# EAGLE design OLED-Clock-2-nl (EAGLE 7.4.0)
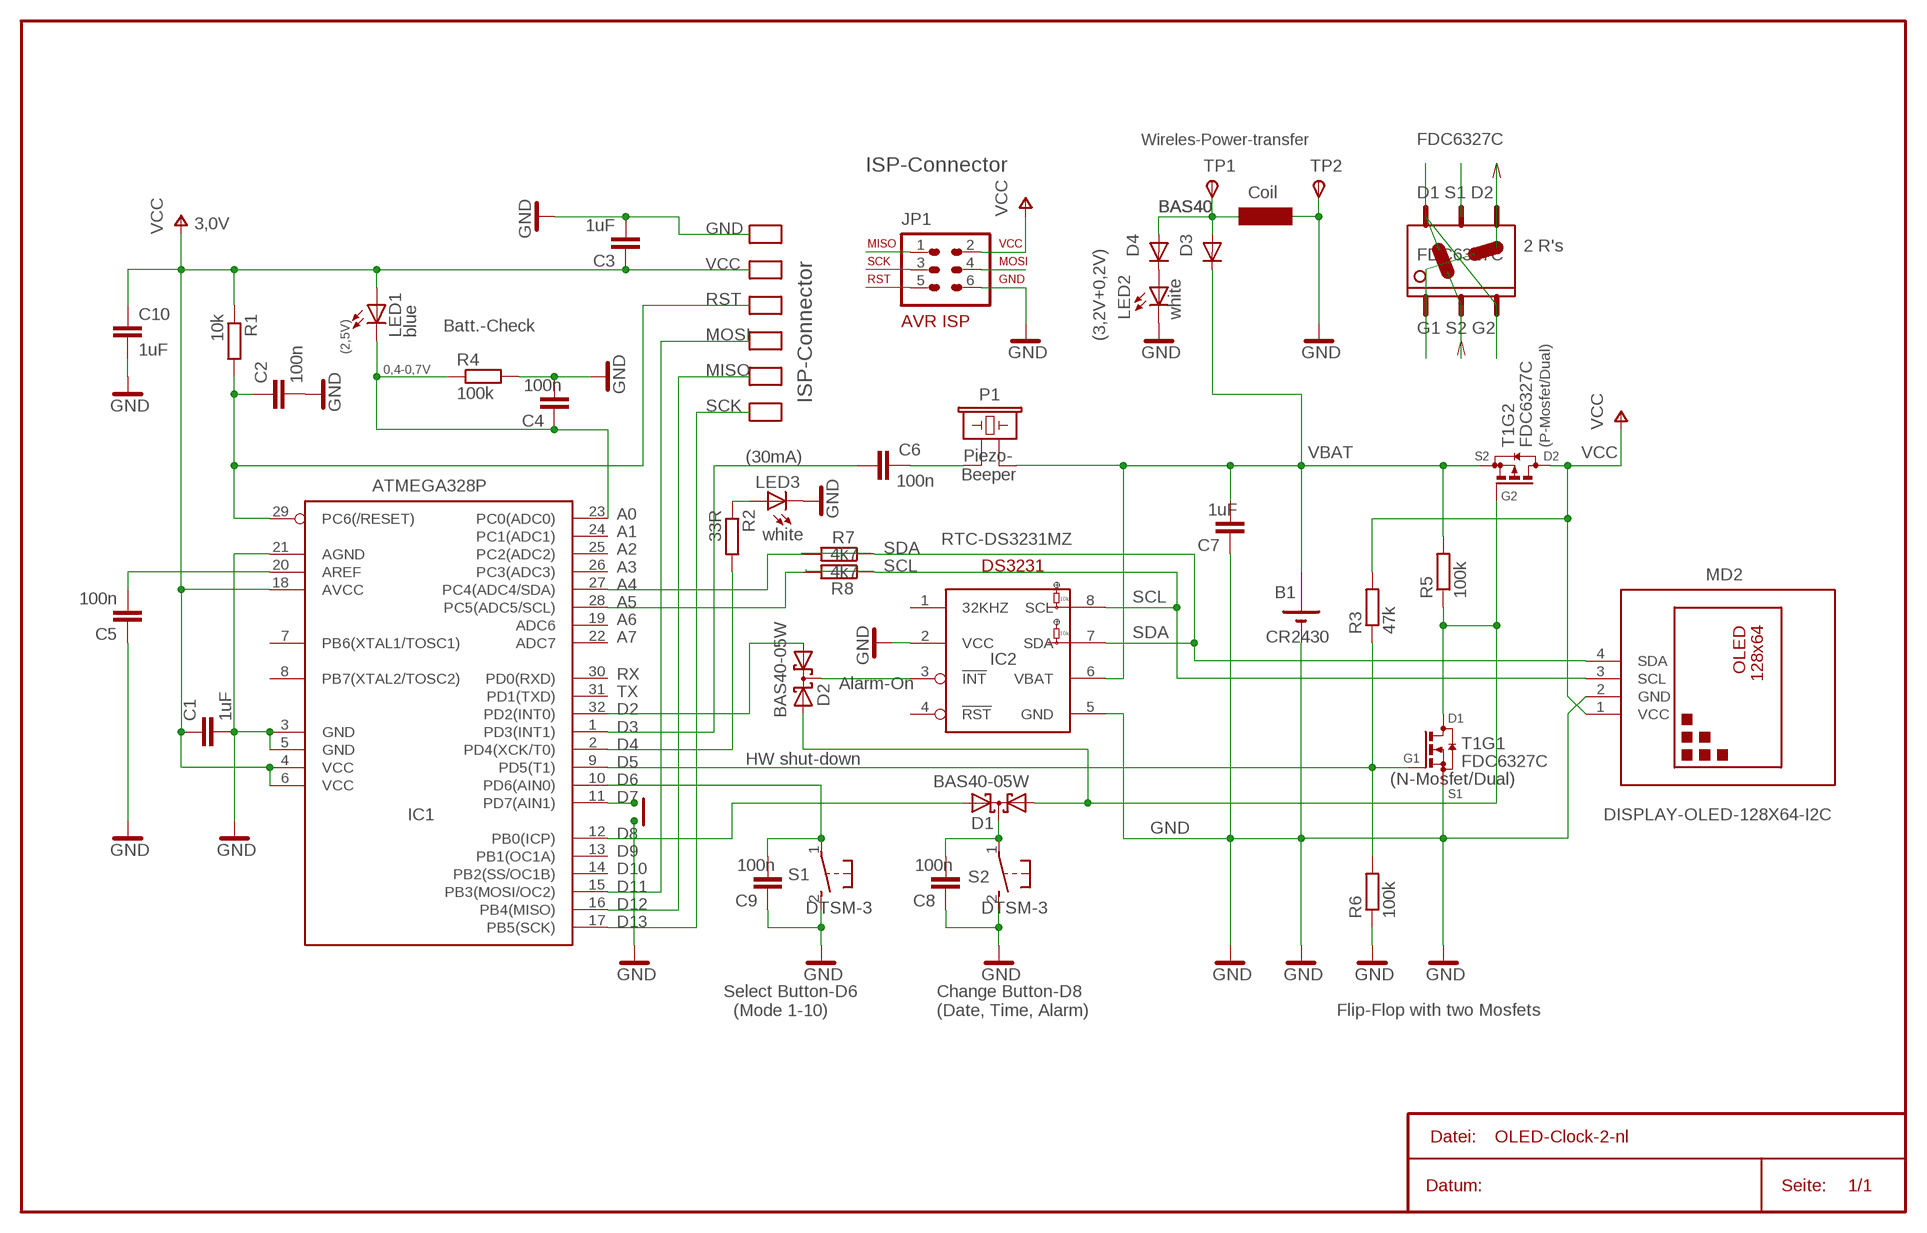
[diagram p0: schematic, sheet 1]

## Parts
C1  1uF  C-EUC0603  [C0603]
C2  100n  C-EUC0603  [C0603]
C3  1uF  C-EUC0603  [C0603]
C4  100n  C-EUC0603  [C0603]
C5  100n  C-EUC0603  [C0603]
C6  100n  C-EUC0805W  [C0805W]
C7  1uF  C-EUC0603  [C0603]
C8  100n  C-EUC0603  [C0603]
C9  100n  C-EUC0603  [C0603]
C10  1uF  C-EUC0603  [C0603]
D1  BAS40-05W  BAS40-05  [SOT323-R]
D2  BAS40-05W  BAS40-05  [SOT323-R]
D3  BAS40  DIODE-SOD523  [SOD523]
D4  BAS40  DIODE-SOD523  [SOD523]
IC1  ATMEGA328P  MEGA8-AI  [TQFP32-08]
IC2  DS3231  [SO08]
JP1  AVR-ISP-6  AVR-ISP-6VERT  [AVR-ISP-6]
LED1  blue  LEDCHIPLED_0805  [CHIPLED_0805]
LED2  white  LEDCHIPLED_0603  [CHIPLED_0603]
LED3  white  LEDCHIPLED_1206  [CHIPLED_1206]
MD2  DISPLAY-OLED-128X64-I2C  [DISPLAY-OLED-128X64-I2C]
R1  10k  R-EU_R0603  [R0603]
R2  33R  R-EU_R0603  [R0603]
R3  47k  R-EU_R0603  [R0603]
R4  100k  R-EU_R0603  [R0603]
R5  100k  R-EU_R0603  [R0603]
R6  100k  R-EU_R0603  [R0603]
R7  4k7  R-EU_R0402  [R0402]
R8  4k7  R-EU_R0402  [R0402]
S1  DTSM-3  [DTSM-3]
S2  DTSM-3  [DTSM-3]
T1  FDC6327C  NP_MOSFET_SOT23-6  [SOT23-6]
TP1  TPSB1,27  [B1,27]
TP2  TPSB1,27  [B1,27]

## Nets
BEEP: C6.1 IC1.1(PD3(INT1))
GND: C1.2 C2.2 C3.2 C4.2 C5.1 C7.1 C8.1 C9.1 C10.2 IC1.3(GND) IC1.5(GND) IC1.21(AGND) IC2.2(VCC) IC2.5(GND) JP1.6 LED2.C LED3.C MD2.2(GND) R4.2 R6.1 S1.2 S2.2 T1.5(S) TP2.TP(PP)
MISO: IC1.16(PB4(MISO)) JP1.1
MOSI: IC1.15(PB3(MOSI/OC2)) JP1.4
N$1: D1.1(A1) D2.2(A2) R5.1 T1.3(G) T1.6(D)
N$2: C9.2 IC1.10(PD6(AIN0)) S1.1
N$5: C6.2
N$6: C8.2 D1.3(C) S2.1
N$7: IC1.11(PD7(AIN1))
N$12: IC1.28(PC5(ADC5/SCL)) R8.2
N$13: C4.1 IC1.23(PC0(ADC0)) LED1.C R4.1
N$16: D1.2(A2) IC1.12(PB0(ICP))
N$21: D2.3(C) IC2.3(!INT)
N$22: LED3.A R2.1
N$23: IC1.2(PD4(XCK/T0)) R2.2
N$25: D3.A D4.A TP1.TP(PP)
N$26: IC1.9(PD5(T1)) R3.1 R6.2 T1.1(G)
N$29: D4.C LED2.A
N$32: C5.2 IC1.20(AREF)
N$33: D2.1(A1) IC1.32(PD2(INT0))
N$34: IC1.27(PC4(ADC4/SDA)) R7.2
RST: C2.1 IC1.29(PC6(/RESET)) JP1.5 R1.2
SCK: IC1.17(PB5(SCK)) JP1.3
SCL: IC2.8(SCL) MD2.3(SCL) R8.1
SDA: IC2.7(SDA) MD2.4(SDA) R7.1
VBAT: C7.2 D3.C IC2.6(VBAT) R5.2 T1.2(S)
VCC: C1.1 C3.1 C10.1 IC1.4(VCC) IC1.6(VCC) IC1.18(AVCC) JP1.2 LED1.A MD2.1(VCC) R1.1 R3.2 T1.4(D)
Unconnected: IC1.7(PB6(XTAL1/TOSC1)) IC1.8(PB7(XTAL2/TOSC2)) IC1.13(PB1(OC1A)) IC1.14(PB2(SS/OC1B)) IC1.19(ADC6) IC1.22(ADC7) IC1.24(PC1(ADC1)) IC1.25(PC2(ADC2)) IC1.26(PC3(ADC3)) IC1.30(PD0(RXD)) IC1.31(PD1(TXD)) IC2.1(32KHZ) IC2.4(!RST)

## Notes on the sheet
- Wireles-Power-transfer | FDC6327C
- ISP-Connector
- Coil | D1 S1 D2
- 3,0V
- 2 R's
- FDC6327C
- Batt.-Check | G1 S2 G2
- (3,2V+0,2V)
- (2,5V)
- 0,4-0,7V
- ISP-Connector | P1
- (P-Mosfet/Dual)
- (30mA) | Piezo- | S2 | D2
- Beeper
- G2
- RTC-DS3231MZ
- +
- B1
- 10k
- +
- 10k
- A0
  A1
  A2
  A3
  A4
  A5
  A6
  A7
- CR2430
- IC2
- Alarm-On
- D1
- HW shut-down | G1
- (N-Mosfet/Dual)
- S1
- RX
  TX
  D2
  D3
  D4
  D5
  D6
  D7
- D8
  D9
  D10
  D11
  D12
  D13
- Select Button-D6
    (Mode 1-10)
- Change Button-D8
  (Date, Time, Alarm)
- Flip-Flop with two Mosfets

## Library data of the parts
C1-C10 = rcl1:C-EU: CAPACITOR, European symbol
D1 D2 = diode1:BAS40-05: Silicon Schottky Diodes General-purpose diode for high-speed switching
D3 D4 = diode1:DIODE-: DIODE
IC1 = avr-7:MEGA8: MICROCONTROLLER 8 Kbytes FLASH 1 kbytes SRAM 512 bytes EEPROM USART 6-channel 10 bit ADC 2-channel 8 bit ADC
IC2 = DS3231:DS3231
JP1 = avr-7:AVR-ISP-6: AVR ISP-6 Serial Programming Header
LED1-LED3 = led:LED: LED
MD2 = diy-modules:DISPLAY-OLED-128X64-I2C: 128x64 Dot Matrix OLED Module based on SSD1306 chip Variant with I2C interface More details available here: http://www.instructables.com/id/Monochrome-096-i2c-OLED-display-with-arduino-SSD13/ SSD1306 datasheet: https://cdn-shop.adafruit.com/datasheets/SSD1306.pdf Click here to find device on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
R1-R8 = rcl:R-EU_: RESISTOR, European symbol
S1 S2 = switch-tact:DTSM-3
T1 = transistor-small-signal:NP_MOSFET_SOT23-6: Dual N- & P-Channel Mosfet 20V / ~2A / ~1W / ~100mO / SOT23-6
TP1 TP2 = testpad-1:TPS: TEST PIN

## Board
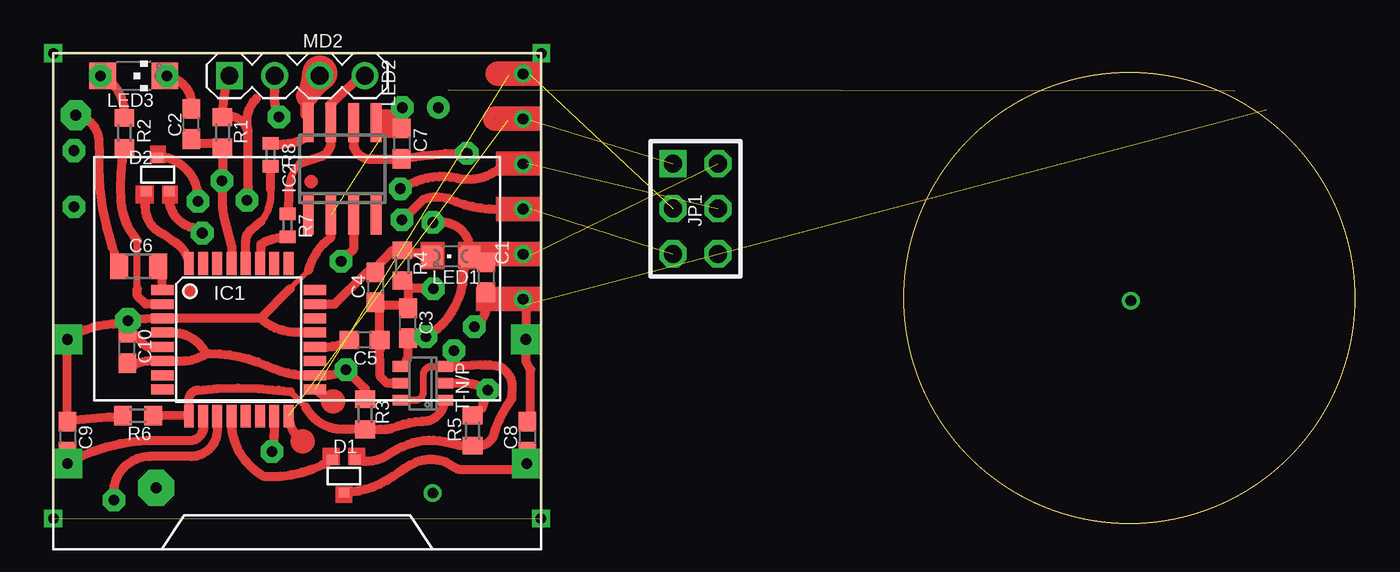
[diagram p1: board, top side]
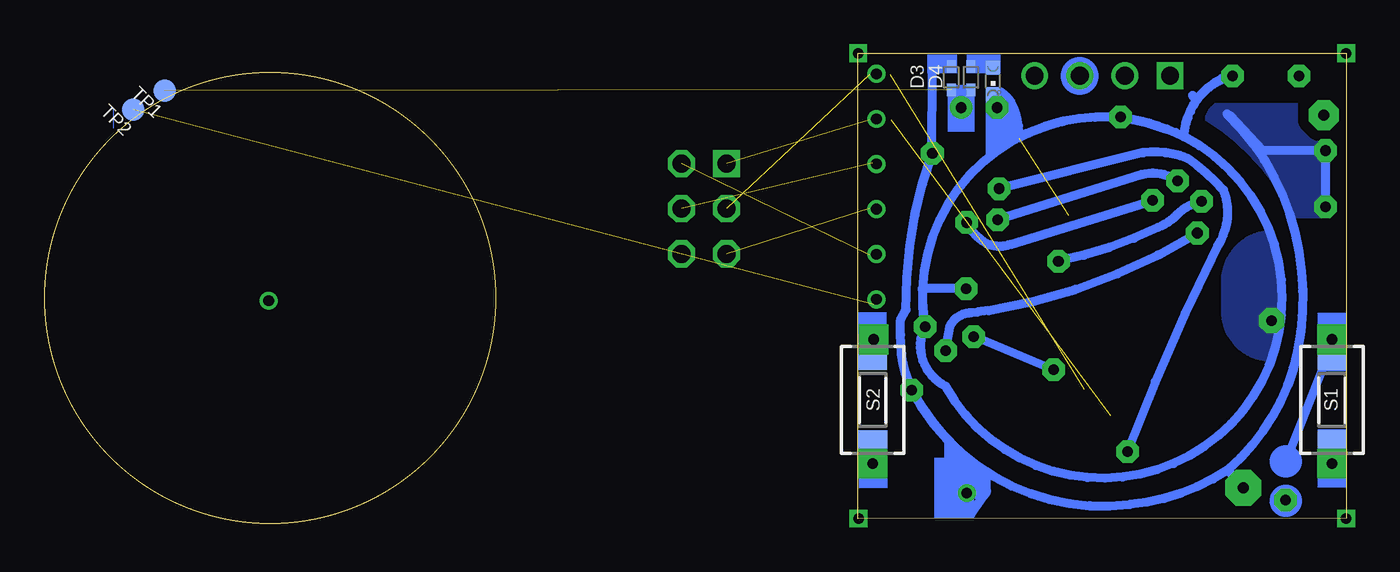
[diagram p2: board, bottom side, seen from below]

Size 73.26 x 26.47 mm. Coordinates in mm from the lower left corner, seen from the top.
Outline: 27.46,0.26 27.46,26.47 0,26.47 0,0.28 27.46,0.26
Outline: circle at 60.56,12.7 radius 12.7
Copper layers (1*16): Top 0.035mm / dielectric 1.5mm / Bottom 0.035mm
Design rules "default": minimum track width 10mil, minimum drill 24mil, track to track 8mil, track to pad 8mil, pad to pad 8mil, via to via 8mil, smd to smd 8mil, copper to edge 40mil, drill to drill 8mil, minimum pad ring 10mil, minimum via ring 8mil, stop-mask expansion 4mil, vias tented up to drill 0mil, thermal gap 10mil

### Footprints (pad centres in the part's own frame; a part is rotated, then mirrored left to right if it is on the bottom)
C0603 = smd 1.1 x 1: 1 -0.85,0; 2 0.85,0
C0805W = smd 1.016 x 1.422: 1 -1.092,0; 2 1.092,0
SOT323-R = smd 0.6 x 0.55: 1 -0.65,-0.925; 2 0.65,-0.925; 3 0,0.925
SOD523 = smd 0.7 x 0.5: A 0.7,0; C -0.6,0
TQFP32-08 = smd 1.27 x 0.559: 1 -4.293,2.8; 2 -4.293,2; 3 -4.293,1.2; 4 -4.293,0.4; 5 -4.293,-0.4; 6 -4.293,-1.2; 7 -4.293,-2; 8 -4.293,-2.8; 17 4.293,-2.8; 18 4.293,-2; 19 4.293,-1.2; 20 4.293,-0.4; 21 4.293,0.4; 22 4.293,1.2; 23 4.293,2; 24 4.293,2.8 | smd 0.559 x 1.27: 9 -2.8,-4.293; 10 -2,-4.293; 11 -1.2,-4.293; 12 -0.4,-4.293; 13 0.4,-4.293; 14 1.2,-4.293; 15 2,-4.293; 16 2.8,-4.293; 25 2.8,4.293; 26 2,4.293; 27 1.2,4.293; 28 0.4,4.293; 29 -0.4,4.293; 30 -1.2,4.293; 31 -2,4.293; 32 -2.8,4.293
SO08 = smd 0.6 x 2.2: 1 -1.905,-2.6; 2 -0.635,-2.6; 3 0.635,-2.6; 4 1.905,-2.6; 5 1.905,2.6; 6 0.635,2.6; 7 -0.635,2.6; 8 -1.905,2.6
AVR-ISP-6 = drill 1.016 square: 1 -2.54,-1.27 | drill 1.016 octagon: 2 -2.54,1.27; 3 0,-1.27; 4 0,1.27; 5 2.54,-1.27; 6 2.54,1.27
CHIPLED_0805 = smd 1.2 x 1.2: A 0,-1.05; C 0,1.05
CHIPLED_0603 = smd 0.8 x 0.8: A 0,-0.75; C 0,0.75
CHIPLED_1206 = smd 1.5 x 1.5: A 0,-1.75; C 0,1.75
DISPLAY-OLED-128X64-I2C = drill 1 square: 1 -3.81,12.7 | drill 1: 2 -1.27,12.7; 3 1.27,12.7; 4 3.81,12.7
R0603 = smd 1 x 1.1: 1 -0.85,0; 2 0.85,0
R0402 = smd 0.7 x 0.9: 1 -0.65,0; 2 0.65,0
DTSM-3 = smd 2 x 1.6: 1 -2.7,0; 2 2.7,0
SOT23-6 = smd 0.6 x 1: 1 -0.95,-1.2; 2 0,-1.2; 3 0.95,-1.2; 4 0.95,1.2; 5 0,1.2; 6 -0.95,1.2
B1,27 = smd 1.27 x 1.27: TP 0,0

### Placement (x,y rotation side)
C1  24.36,13.86 270 top
C2  7.77,22.49 90 top
C3  19.96,11.28 90 top
C4  18.13,13.3 270 top
C5  17.51,10.33 180 top
C6  4.8,14.49 180 top
C7  19.61,21.39 270 top
C8  26.67,4.88 270 top
C9  0.79,4.88 270 top
C10  4.17,9.88 90 top
D1  16.35,2.66 180 top
D2  5.87,19.65 0 top
D3  22.23,25.12 270 bottom
D4  21.11,25.12 270 bottom
IC1  10.43,10.34 0 top
IC2  16.26,19.97 0 top
JP1  36.14,17.72 270 top
LED1  22.37,15.05 90 top
LED2  19.88,24.91 180 bottom
LED3  4.52,25.2 270 top
MD2  13.72,12.51 0 top
R1  9.53,22.03 270 top
R2  4.01,21.99 270 top
R3  17.55,6.15 90 top
R4  19.63,14.53 270 top
R5  23.59,5.23 90 top
R6  4.76,6.07 0 top
R7  13.18,16.79 270 top
R8  12.22,20.76 270 top
S1  0.79,6.95 90 bottom
S2  26.64,6.95 90 bottom
T1  20.8,7.89 90 top
TP1  66.5,24.37 135 bottom
TP2  68.28,23.31 135 bottom

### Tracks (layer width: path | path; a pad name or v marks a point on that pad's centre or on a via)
BEEP
  Top 0.508: IC1.1 6.14,14.8 C6.1
GND  (via drill 0.6 pad 0.81, 0.6 pad 1.27, 0.6 pad 1.42, 0.6 pad 1.68)  (3 unrouted)
  Top 0.305: 13.34,13.22 14.37,14.25
  Top 0.508: 26.37,12.56 26.27,12.66 24.47,12.66 C1.2 24.36,12.33 arc-63 v23.69,11.07 | 26.37,12.56 26.59,12.34 v26.59,10.36 26.59,9.13 26.87,8.65 26.87,5.41 C8.1 | 18.4,9.82 C5.1 | T1.5 18.78,7.89 18.4,8.27 C5.1 | 19.86,11.97 C3.2 | 11.67,11.55 11.66,11.54 IC1.3 5.56,11.55 v4.2,11.42 | 11.67,11.55 13.34,13.22 | 14.37,14.25 arc-40 15.62,16.1 IC2.2 | 0.79,5.44 C9.1 | C9.1 v0.79,10.36 arc-36 3.76,11.23 v4.2,11.42 | IC1.21 13.73,10.76 arc-44 11.67,11.55 | IC2.5 C7.1 19.53,22.19 arc-17 v19.64,23.42 | v26.43,12.62 26.37,12.56 | 19.96,11.87 C3.2 | R4.2 19.52,13.57 19.96,13.57 19.96,13.22 | 19.96,13.22 C3.2 | v21.39,13.22 19.96,13.22 | C3.2 19.96,12.32 | 18.43,12.31 C4.2 | C5.1 18.36,12.25 18.43,12.31 | 18.43,12.31 19.77,12.31 C3.2 | v12.7,22.9 arc-28 12.46,24.33 MD2.2 v12.46,25.2 | C2.2 7.81,23.74 arc70 v6.39,25.2 LED3.C | C10.2 3.89,11.2 v4.2,11.42 | IC1.5 5.26,9.94 4.24,10.97 v4.2,11.42 | R6.1 3.81,5.97 3.06,5.97 0.83,5.77 C9.1
  Bottom 0.508: S2.2 26.59,9.51 v26.59,10.36 | S1.2 0.79,10.12 | 0.79,10.12 v0.79,10.36 | v21.39,13.22 23.85,13.22 arc-11 v23.69,11.07 23.76,11.11 23.76,11.06 | 3.65,11.71 arc-195 23.73,11.15 23.76,11.06 | 23.76,11.06 23.89,10.64 arc-78 22.54,7.74 arc-146 3.65,11.79 arc-90 3.73,11.54 v4.2,11.42 | 10.6,22.38 arc-46 18.41,21.71 arc-30 18.85,23.69 arc-31 19.45,24.29 v19.64,23.42 19.88,24.01 LED2.C | 0.79,10.12 3.41,3.45 | v12.7,22.9 12.62,22.82 arc14 10.6,22.38 | 10.6,22.38 arc10 9.13,21.79 arc65 6.67,25.2 v6.39,25.2 arc-41 8.41,23.85 8.65,24.09
  pour Bottom: 4.17,16.39 arc-84 6.91,13.93 6.91,11.79 arc-90 4.13,9.25 arc-38
MISO  (via drill 0.6 pad 0.81)  (2 unrouted)
  Top 0.508: 25.58,22.72 26.47,22.72 | 26.47,22.72 26.85,22.72 | IC1.16 13.26,5.99 arc50 13.93,4.72 | v26.43,22.78 26.43,22.76 26.47,22.72
MOSI  (via drill 0.6 pad 0.81, 0.6 pad 1.27)  (1 unrouted)
  Top 0.508: IC1.15 12.43,5.49 arc-11 v12.3,4.05 | v19.53,18.85 20.4,19.25 arc-32 22.7,19.45 arc44 24.84,19.8 arc-38 v26.43,20.24 26.63,20.24 26.67,20.28
  Bottom 0.508: v19.53,18.85 11.43,20.88 arc29 8.93,20.56 arc13 6.91,18.77 arc53 7.22,15.64 arc-6 v12.3,4.05
N$1  (via drill 0.6 pad 1.27)
  Top 0.406: T1.6 20.39,6.94 arc86 20.82,7.36 20.82,8.39 arc-79 21.26,8.84 T1.3
  Top 0.508: 22.62,8.84 T1.3 | 22.62,8.84 22.5,9.12 v22.54,9.72 | D1.1 arc46 18.69,3.77 arc-10 19.68,4.33 arc-44 22.3,4.52 22.88,4.38 R5.1 24.13,4.38 arc51 24.77,4.92 arc-18 25.8,7.02 25.84,7.6 arc68 25.08,8.85 arc16 24.05,8.93 arc1 22.62,8.84 | v8.37,16.35 7.82,16.67 arc-88 D2.2
  Bottom 0.508: v22.54,9.72 22.3,11.07 arc67 21.11,11.87 20.76,11.91 20.12,11.99 arc-22 v8.37,16.35
N$2  (via drill 0.6 pad 1.68)
  Top 0.508: v0.79,3.37 0.87,3.37 0.87,3.29 v0.79,3.37 | v0.79,3.37 C9.2 | IC1.10 8.45,5.64 arc-87 7.86,4.68 5.32,4.68 arc28 v0.79,3.37
  Bottom 0.508: S1.1 v0.79,3.37
N$4  (via drill 0.6)
  other vias: 0,26.47
N$5  (via drill 0.6 pad 1.68)
  Top 0.508: C6.2 arc-27 2.58,21.15 2.58,21.47 arc81 v1.26,22.99
N$6  (via drill 0.6 pad 1.68)
  Top 0.406: C8.2 26.64,4.03 | 26.64,4.03 S2.1 | 26.64,4.03 v26.64,3.37
  Top 0.508: D1.3 arc33 19.12,2.65 arc-12 20.4,3.45 arc-42 22.11,3.45 22.78,3.06 26.43,3.06 v26.64,3.37
  Bottom 0.406: S2.1 v26.64,3.37
N$7  (via drill 0.6 pad 1.27)
  Top 0.508: IC1.11 arc-23 9.13,4.72 arc-67 7.78,3.77 5.4,3.77 arc100 v3.41,1.31
N$9  (via drill 0.6)
  other vias: 27.46,26.47
N$10  (via drill 0.6)
  other vias: 27.44,0.28
N$11  (via drill 0.6)
  other vias: 0,0.28
N$12
  Top 0.406: 11.67,16.99 arc52 12.22,18.85
  Top 0.508: IC1.28 10.84,15.87 arc-53 11.15,16.55 11.67,16.99 | 12.22,18.85 R8.2
N$13
  Top 0.508: LED1.C 21.32,15.13 | IC1.23 15.84,12.34 17.65,14.15 C4.1 18.1,14.15 18.1,14.33 19.12,15.38 R4.1 19.63,15.24 21.04,15.24 21.04,15.13 LED1.C | LED1.C | 21.2,15.05 LED1.C
N$16
  Top 0.508: IC1.12 10.03,5.49 arc55 11.83,2.66 12.78,2.66 arc24 D1.2
N$21  (via drill 0.6 pad 1.27)
  Top 0.508: IC2.3 16.89,15.43 v16.19,14.76 | D2.3 6.02,20.68 arc-87 v8.14,18.14
  Bottom 0.508: v8.14,18.14 arc-35 9.53,17.38 arc25 10.6,16.67 arc14 v16.19,14.76
N$22  (via drill 0.6 pad 1.27)
  Top 0.508: R2.1 arc64 LED3.A v2.66,25.2
N$23
  Top 0.406: 4.72,13.22 4.72,15.91
  Top 0.508: IC1.2 5.2,12.34 4.72,12.82 4.72,13.22 | R2.2 arc14 3.81,18.18 arc34 4.72,15.91
N$24
  Top 0.406: 14.68,23.93 arc-13 15.56,24.8
N$25  (via drill 0.6 pad 1.27)  (1 unrouted)
  Bottom 0.508: D4.A D3.A 21.67,24.41 v21.67,23.42
N$26
  Top 0.356: 13.34,7.42 14.21,6.55
  Top 0.508: 13.34,7.42 12.66,7.5 arc13 8.14,7.5 arc77 7.62,7.02 IC1.9 7.61,5.83 7.62,5.83 7.52,6.12 R6.2 | 14.21,6.55 arc60 16.17,5.3 R3.1 18.4,5.3 arc19 19.05,5.36 arc-19 20.74,5.75 arc93 T1.1
N$27
  Top 0.406: 13.89,24.17 arc23 14.21,25.44
N$29
  Bottom 0.508: D4.C 20.1,25.72 LED2.A
N$30  (via drill 0.6)
  other vias: 60.64,12.54
N$31
  Bottom 0: 69.37,22.26 69.37,23.38
N$32
  Top 0.508: IC1.20 arc30 16.67,10.26 C5.2
N$33
  Top 0.508: IC1.32 arc56 6.71,15.91 6.15,16.31 arc-93 5.34,18.6 D2.1
N$34
  Top 0.508: R7.2 arc28 11.67,15.72 IC1.27
RST  (via drill 0.6 pad 0.81, 0.6 pad 1.27)  (1 unrouted)
  Top 0.508: IC1.29 10.03,15.65 9.6,17.26 arc-11 9.53,18.89 v9.48,19.29 9.53,19.33 R1.2 9.31,21.39 7.98,21.39 C2.1 | v19.61,17.11 19.68,17.11 20.84,18.26 arc-35 22.23,18.3 arc25 25,17.7 v26.43,17.7 26.83,17.74
  Bottom 0.508: v9.48,19.29 arc-51 11.51,19.65 v19.61,17.11
SCK  (via drill 0.6 pad 0.81)  (2 unrouted)
  Top 0.508: IC1.17 15.68,6.83 | 25.64,25.28 26.43,25.28 | 26.43,25.28 26.83,25.28 | v26.43,25.32 26.43,25.28
SCL  (via drill 0.6 pad 1.27)
  Top 0.508: MD2.3 v15,25.2 | 14.3,23.19 14.28,23.06 IC2.8 14.33,21.95 14.21,21.71 arc-39 R8.1
  Top 0.762: 14.28,24.06 14.28,23.06
  Top 1.27: MD2.3 14.28,24.06
SDA  (via drill 0.6 pad 1.27)
  Top 0.406: 13.89,20.28 arc50 13.26,18.77
  Top 0.508: v17.54,25.2 MD2.4 17.31,25.21 15.55,23.56 IC2.7 15.62,21.32 arc-48 15.1,20.68 13.89,20.28 | 13.26,18.77 13.26,18.3 R7.1
VBAT  (via drill 0.6 pad 0.81, 0.6 pad 1.27, 0.6 pad 2.03)
  Top 0.508: T1.2 22.79,7.89 arc-29 24.29,7.62 v24.45,7.5 24.14,6.48 R5.2 | IC2.6 16.89,21.24 arc80 18.02,20.52 19.17,20.52 C7.2 arc-12 v23.29,20.84
  Bottom 0.508: v24.45,7.5 arc24 25.08,10.64 25.08,11.47 24.77,12.03 arc21 v23.29,20.84 23.34,20.95 23.32,25.45 23.05,25.72 D3.C | 6.71,23.06 arc36 2.66,15.32 arc21 2.74,9.68 arc37 6.66,3.02 | v24.45,7.5 arc-70 12.18,1.07 arc-29 6.66,3.02 | 20.31,2.84 arc25 v24.45,7.5 | v5.79,2 6.66,3.02 | 20.32,2.04 v21.35,1.71 20.39,1.57 21.11,0.53 | v1.15,17.82 v1.15,20.99 4.68,20.99 6.55,22.98
  Bottom 0.61: 22.3,4.56 22.3,2.84 20.31,2.84 20.31,1.73 20.32,2.04
  pour Bottom (isolate 0.61): 7.86,23.53 7.86,22.82 arc32 2.9,17.34 0.24,17.34 0.24,21.27 2.62,23.53
VCC  (via drill 0.6 pad 0.81, 0.6 pad 1.27)  (1 unrouted)
  Top 0.508: R3.2 17.55,7.58 v16.47,8.65 16.38,8.58 arc-27 IC1.18 14,8.34 arc-20 11.99,8.89 arc25 8.81,9.56 8.59,9.55 | T1.4 arc52 19.96,9.43 C3.1 20.05,10.52 v20.95,10.52 21.27,10.68 arc59 23.1,14.72 LED1.A | 26.39,15.12 24.85,15.12 C1.1 23.68,14.79 LED1.A | 26.39,15.12 26.83,15.12 | IC1.4 6.9,10.74 arc-60 8.59,9.55 | 8.59,9.55 arc-32 7.2,9.14 IC1.6 5.29,9.14 4.64,8.97 4.14,8.97 C10.1 | v26.43,15.16 26.39,15.12 | LED1.A arc107 21.75,16.95 v21.35,16.95 | v10.89,18.19 10.95,19.05 10.95,22.07 | 10.95,22.07 arc96 R1.1 arc-17 9.84,25.04 v9.92,25.2 MD2.1 | 11.43,23.93 arc59 10.95,22.15 10.95,22.07
  Bottom 0.508: v16.47,8.65 v20.95,10.52 | v10.89,18.19 18.89,15.72 arc45 20.24,15.76 arc32 v21.35,16.95
(copper drawn outside any net)
  shapes: Bottom area x15, Bottom circle x3, Top area x18, Top circle x8

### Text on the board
tNames: T-N/P
tValues: Board: ~28 x 26,5 mm | Layer: | 1. Beeper (ø24mm) / 2. Batt. (CR2430) / 3. ATmega-Board / 4. OLED-Display | (GND VCC) | Coil with / 30 loops / Cu 0.1mm | Beeper+ | Beeper- | GND | SCL / SDA / VBat / GND | GND | VBAT | RTC-DS3231 | MISO | VCC | VBAT | SCK | MOSI | 32kHz / VCC / INT/SQW / !RST | RM2,54mm | Wireless-Power-transfer | D2 | RST | A5 | A4 | RST | GND | D3 | D4 | A0 | A1 | SCK / MISO / MOSI / RST / VCC / GND | (von oben) | GND | GND | AREF | VCC | X1 | X2 | SCK | VCC | !! Buttons / on Bottom !! | D5 | D6 | D7 | D8 | MOSI | MISO | FDC6327C | Select Button | VBAT | Change Button | Reset | VBAT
